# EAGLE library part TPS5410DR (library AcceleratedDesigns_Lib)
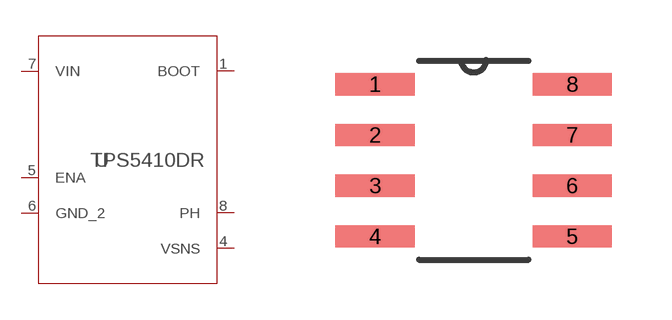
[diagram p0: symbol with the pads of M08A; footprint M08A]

Designator prefix -

## TPS5410DR (DATASHEETURL: httpwww.ti.comproducttps5410; FREQUENCY: 500000.0; IMAX: 1.0; MANUFACTURER_NAME: Texas Instruments; MANUFACTURER_PART_NUMBER: TPS5410DR; MKTG_PACKAGE: TPS5410; NSID: TPS5410D; PACKAGE: TPS5410; VENDOR: Texas Instruments)  [M08A]
1  BOOT  pas
4  VSNS  pas
5  ENA  pas
6  GND_2  pas
7  VIN  pas
8  PH  pas

## Footprint M08A (pad centres in mm)
smd 1.981 x 0.559: 1 -2.464,1.905; 2 -2.464,0.635; 3 -2.464,-0.635; 4 -2.464,-1.905; 5 2.464,-1.905; 6 2.464,-0.635; 7 2.464,0.635; 8 2.464,1.905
